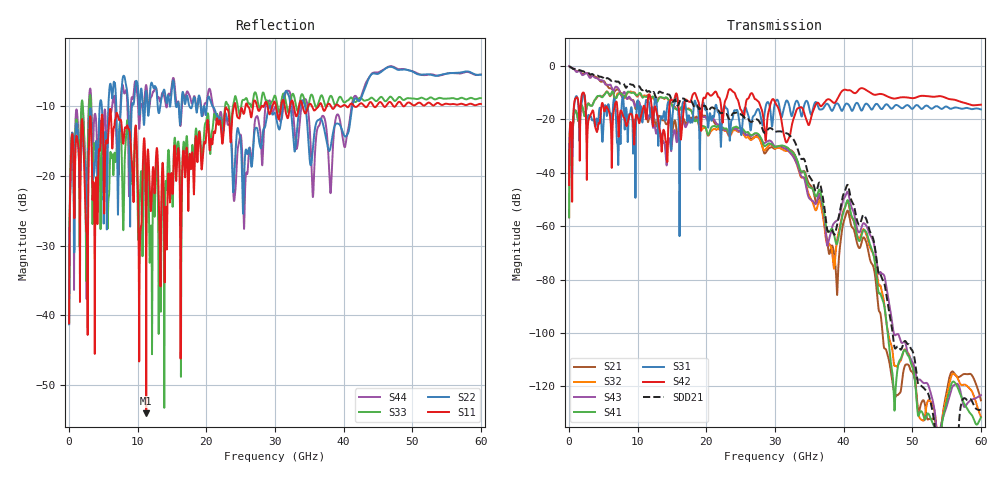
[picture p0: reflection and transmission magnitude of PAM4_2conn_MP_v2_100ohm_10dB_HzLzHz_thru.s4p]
! Info: Touchstone file created by Circ.  Input file=FAB50GbE_2conn_Midplane_Examax_Topo2_v2_100ohm_10dB_HzLzHz.circ
# Hz S RI R 50
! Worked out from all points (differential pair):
!   6000 points, 10 MHz to 60 GHz, reference 50 ohm
!   strongest paths, dB at 10 MHz, 15.01 GHz, 30.01 GHz, 45.01 GHz, 60 GHz:
!     S42: -44.6, -12.9, -13.6, -10.6, -14.5
!     S31: -44.7, -21.3, -13.8, -14.6, -16.3
!     S41: -56.7, -14.8, -30.4, -83.5, -131.7
!     S43: -0.1, -28.4, -30.2, -76.5, -123.3
!     S32: -56.7, -14.6, -30.8, -80.7, -131.5
!     S21: -0.1, -24.9, -31.0, -89.3, -125.2
!   taken as a pair (ports 3,1 in; 4,2 out), SDD21 dB: -0.1, -13.2, -24.7, -76.6, -128.6
!   lowest |S11| = -54.1 dB at 11.24 GHz (marker M1), VSWR 1.00, Z = 50.2 + j0.0333 ohm
!   |S11| at or under -10 dB: start of sweep to 24.02 GHz; 24.28 GHz to 25.7 GHz (1.416 GHz wide, 5.67 % of centre); 35.4 GHz to 36.35 GHz (955.4 MHz wide, 2.66 % of centre)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
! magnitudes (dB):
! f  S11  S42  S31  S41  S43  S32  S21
! 10 MHz  -41.2  -44.6  -44.7  -56.7  -0.1  -56.7  -0.1
! 930 MHz  -16.6  -12.2  -11.9  -16.7  -1.9  -16.6  -1.7
! 11.24 GHz  -54.1  -20.0  -12.7  -11.6  -16.8  -11.5  -16.4
! 32.48 GHz  -9.2  -21.9  -18.7  -32.2  -33.4  -33.0  -31.8
! 38.99 GHz  -9.8  -12.9  -14.0  -66.8  -58.0  -66.3  -82.7
! 40.55 GHz  -10.1  -9.1  -14.2  -50.3  -47.1  -50.8  -54.2
! 60 GHz  -9.7  -14.5  -16.3  -131.7  -123.3  -131.5  -125.2
